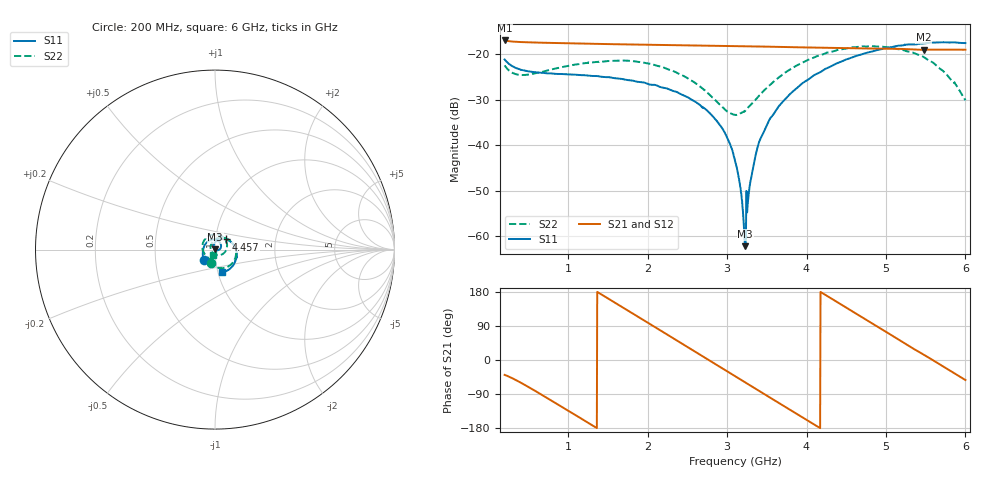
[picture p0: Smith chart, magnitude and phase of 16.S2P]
!Agilent Technologies,E5071C,MY46316741,A.11.02
!Date: Fri Apr 15 16:22:40 2022
!Data & Calibration Information:
!Freq	S11:SOLT2(ON)	S21:SOLT2(ON)	S12:SOLT2(ON)	S22:SOLT2(ON)
!PortZ  Port1:50+j0  Port2:50+j0
!Above PortZ is port z conversion or system Z0 setting when saving the data.
!When reading, reference impedance value at option line is always used.
# Hz S dB R 50
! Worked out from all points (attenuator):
!   1200 points, 200 MHz to 6 GHz, reference 50 ohm
!   highest |S21| = -16.93 dB at 200 MHz (marker M1); lowest = -19.0 dB at 5.478 GHz (marker M2)
!   lowest |S11| = -62.2 dB at 3.228 GHz (marker M3), VSWR 1.00, Z = 50.1 + j0.0593 ohm
!   |S11| at or under -10 dB: start of sweep to end of sweep
!   |S22| runs from -33.3 to -18.2 dB; largest |S21 - S12| = 0.00056
!   S11 on the Smith chart (normalised r, x): 200 MHz: 0.87, -0.11; 4.457 GHz: 1.13, +0.13; 6 GHz: 1.05, -0.27
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2e8  -21.10 -136.6  -16.93 -39.3  -16.93 -39.3  -22.41 -105.9
4.418682e8  -23.51 -177.2  -17.31 -64.3  -17.31 -64.3  -24.53 -137.8
1.167473e9  -24.56 118.4  -17.61 -155.0  -17.61 -155.0  -22.04 139.9
1.588324e9  -25.24 86.7  -17.76 151.3  -17.76 151.3  -21.40 93.4
2.134946e9  -26.99 46.2  -17.90 81.4  -17.90 81.5  -22.56 27.7
2.768641e9  -32.68 -2.9  -18.05 -0.0  -18.05 0.1  -28.68 -59.3
2.966972e9  -37.08 -17.4  -18.12 -25.5  -18.12 -25.5  -31.96 -104.1
3.102419e9  -43.49 -24.2  -18.16 -42.9  -18.16 -42.8  -33.32 -146.4
3.160467e9  -48.37 -30.4  -18.18 -50.4  -18.18 -50.3  -33.05 -166.1
3.208841e9  -56.84 -10.9  -18.19 -56.6  -18.20 -56.5  -32.60 178.7
3.22819e9  -62.18 49.6  -18.20 -59.1  -18.20 -59.0  -32.41 172.8
3.24754e9  -50.11 145.2  -18.21 -61.6  -18.21 -61.4  -32.02 166.6
3.271726e9  -50.83 127.8  -18.21 -64.7  -18.22 -64.6  -31.56 160.0
3.363636e9  -41.87 122.9  -18.24 -76.5  -18.24 -76.4  -29.88 138.0
3.50392e9  -35.39 115.5  -18.29 -94.4  -18.29 -94.3  -27.29 112.4
3.697415e9  -30.48 101.8  -18.36 -119.2  -18.36 -119.1  -24.46 84.7
4.069892e9  -24.90 71.8  -18.50 -166.8  -18.49 -166.7  -20.86 41.3
4.456881e9  -21.45 41.8  -18.59 143.8  -18.59 143.9  -18.83 2.6
5.037364e9  -18.47 -2.6  -18.75 69.6  -18.76 69.7  -18.49 -52.7
5.477565e9  -17.59 -35.0  -18.99 13.8  -18.99 13.9  -20.60 -90.3
5.74362e9  -17.34 -54.2  -18.95 -19.9  -18.96 -19.8  -24.01 -109.0
6e9  -17.51 -72.6  -18.96 -52.8  -18.98 -52.6  -30.11 -111.6
